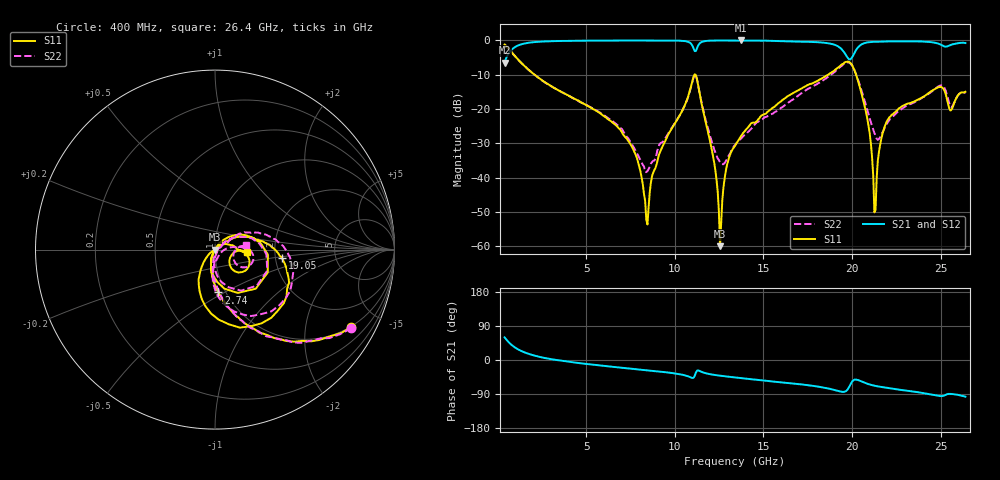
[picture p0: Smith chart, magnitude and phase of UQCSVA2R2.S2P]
!  Part Number  UQCSVA2R2  Mounting Orientation: Horizontal
!  Description: Ultra Low ESR Microwave capacitors
!  Application: Coupling, Bypass, Tuning, DC Block
!  Filters, Matching
# GHZ S DB R 50
! Freq  |S11|  S11 Ph  |S21|  S21 Ph  |S12|  S12 Ph  |S22|  S22 Ph
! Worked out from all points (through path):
!   401 points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, 400 MHz to 26.4 GHz, reference 50 ohm
!   highest |S21| = 0.00 dB at 13.72 GHz (marker M1); lowest = -6.4 dB at 400 MHz (marker M2)
!   group delay of S21, straight-line fit = 12.1 ps
!   lowest |S11| = -60.0 dB at 12.55 GHz (marker M3), VSWR 1.00, Z = 50 - j0.0918 ohm
!   |S11| at or under -10 dB: 2.092 GHz to 11.11 GHz (9.022 GHz wide, 137 % of centre); 11.17 GHz to 18.65 GHz (7.477 GHz wide, 50.1 % of centre); 20.23 GHz to end of sweep
!   |S22| runs from -38.4 to -1.1 dB; largest |S21 - S12| = 0.0079
!   S11 on the Smith chart (normalised r, x): 400 MHz: 0.97, -3.53; 2.74 GHz: 0.93, -0.47; 19.05 GHz: 2.18, -0.23; 26.4 GHz: 1.43, -0.04
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0.4  -1.17 -29.6  -6.43 59.8  -6.44 59.7  -1.15 -30.0
1.31  -6.36 -64.7  -1.17 24.4  -1.18 24.6  -6.40 -65.6
2.74  -12.42 -85.4  -0.28 4.6  -0.29 4.8  -12.48 -84.3
4.755  -18.18 -99.5  -0.07 -8.9  -0.07 -8.9  -18.15 -95.1
7.485  -30.10 -115.9  -0.01 -22.7  -0.01 -22.6  -29.53 -92.7
8.395  -52.25 -162.7  -0.02 -27.1  -0.02 -27.0  -38.41 -29.8
9.11  -33.28 59.5  -0.04 -30.5  -0.04 -30.4  -30.61 29.4
11.19  -10.04 -43.8  -3.09 -33.4  -3.08 -33.5  -10.24 -40.7
12.165  -33.90 -116.3  -0.03 -38.9  -0.04 -38.8  -30.72 -80.5
12.555  -59.99 -66.3  -0.01 -41.4  -0.01 -41.3  -35.52 -44.4
12.945  -36.37 53.3  -0.01 -43.6  -0.01 -43.5  -34.67 2.0
13.4  -30.74 45.5  -0.01 -46.0  -0.01 -45.9  -30.50 20.5
13.725  -28.00 44.5  0.00 -47.7  0.00 -47.5  -28.69 25.0
17.755  -12.54 13.2  -0.44 -68.0  -0.42 -67.8  -13.47 26.8
19.055  -8.49 -6.9  -1.32 -79.5  -1.32 -79.6  -9.06 7.1
20.225  -9.89 -99.5  -2.85 -51.6  -2.84 -51.6  -9.76 -77.9
20.875  -23.09 -136.0  -0.55 -62.8  -0.54 -62.7  -20.37 -93.8
21.265  -50.12 -142.7  -0.38 -67.8  -0.36 -67.6  -27.01 -68.1
22.11  -22.43 23.4  -0.28 -74.5  -0.27 -74.5  -23.18 5.8
24.905  -13.61 -24.1  -0.98 -94.8  -0.99 -94.8  -13.31 -9.1
25.555  -20.44 -27.0  -1.33 -89.5  -1.32 -89.4  -19.24 -21.7
26.4  -14.96 -4.3  -0.75 -96.7  -0.75 -96.5  -15.20 7.9
